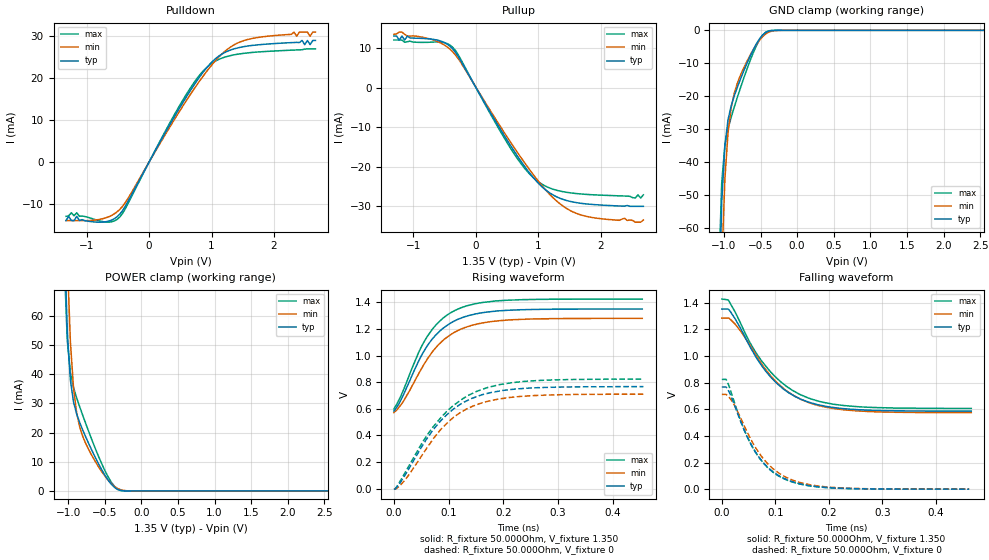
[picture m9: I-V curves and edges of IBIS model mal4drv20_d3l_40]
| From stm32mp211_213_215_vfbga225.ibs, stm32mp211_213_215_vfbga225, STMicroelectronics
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[Model] mal4drv20_d3l_40
Model_type   I/O
Polarity   Non-Inverting
Enable   Active-High
C_comp   1.902pF   1.872pF   1.915pF
C_comp_pullup   928.637fF   913.380fF   944.342fF
C_comp_pulldown   824.069fF   818.585fF   846.427fF
Vinh = 805.000mV
Vinl = 545.000mV
Vmeas = 675.000mV
Vref = 675.000mV
Rref = 50Ohms
Cref = 0pF
[Model Spec]
Vinh   805.000mV   772.000mV   855.000mV
Vinl   545.000mV   512.000mV   595.000mV
Vmeas   675.000mV   642.000mV   725.000mV
Vref   675.000mV   642.000mV   725.000mV
D_overshoot_ampl_h 0.4 NA   NA
D_overshoot_ampl_l 0.4 NA   NA
D_overshoot_area_l 110.000m NA   NA
D_overshoot_area_h 110.000m NA   NA
[Temperature Range]   25.000   125.000   -40.000
[Voltage Range]   1.350V   1.283V   1.425V
[GND Clamp Reference]   0.00V   0.00V   0.00V
[C Comp Corner]
| variable   typ   min   max
C_comp   1.902pF   1.872pF   1.915pF
C_comp_pullup   928.637fF   913.380fF   944.342fF
C_comp_pulldown   824.069fF   818.585fF   846.427fF
[Pulldown Reference]   0.00V   0.00V   0.00V
[POWER Clamp Reference]   1.350V   1.283V   1.425V
[Pullup Reference]   1.350V   1.283V   1.425V
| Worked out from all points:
|   slope of the pulldown table from 0 to 0.203 V, typ, clamps not added: 36.8 ohm
|   slope of the pullup table from 0 to 0.203 V, typ, clamps not added: 36.7 ohm
|   GND clamp passes 1 mA (typ) near -0.45 V on its own axis
|   POWER clamp passes 1 mA (typ) near -0.35 V on its own axis
|   rising waveform, R_fixture 50.000Ohm, V_fixture 1.350: 20-80 % time 66.2ps typ, 71.6ps min, 64ps max; typ from 0.584 V to 1.35 V
|   rising waveform, R_fixture 50.000Ohm, V_fixture 0: 20-80 % time 86.1ps typ, 86.2ps min, 93.2ps max; typ from -0.004 V to 0.767 V
|   falling waveform, R_fixture 50.000Ohm, V_fixture 1.350: 20-80 % time 83.5ps typ, 86.2ps min, 88.4ps max; typ from 1.35 V to 0.586 V
|   falling waveform, R_fixture 50.000Ohm, V_fixture 0: 20-80 % time 63.3ps typ, 68.1ps min, 62ps max; typ from 0.767 V to 0 V
[GND Clamp]
-1.332V   -728mA     -688mA     -718.9mA
-1.074V   -89.22mA   -115mA     -76.03mA
-1.031V   -52.27mA   -71.45mA   -46.39mA
-988mV    -34.98mA   -45.32mA   -35.1mA
-945mV    -27.21mA   -31.15mA   -29.98mA
-902mV    -22.97mA   -23.56mA   -26.45mA
-859.1mV  -19.9mA    -19.1mA    -23.3mA
-773.2mV  -14.75mA   -13.57mA   -17.39mA
-601.4mV  -5.967mA   -5.934mA   -6.902mA
-429.5mV  -634uA     -1.09mA    -554.5uA
-214.8mV  -1.1uA     -11.75uA   -194.3nA
2.663V    35.59nA    706.2nA    31.73nA
[Power Clamp]
-1.313V   833mA      802.3mA    823.6mA
-1.055V   90.5mA     128mA      79.41mA
-1.012V   54.31mA    79.78mA    51.52mA
-969.5mV  37.92mA    51.03mA    40.54mA
-926.6mV  30.49mA    35.21mA    35.43mA
-883.6mV  26.34mA    26.67mA    31.87mA
-840.7mV  23.31mA    21.76mA    28.71mA
-754.8mV  18.2mA     15.96mA    22.74mA
-583mV    9.188mA    8.193mA    11.73mA
-454.1mV  3.709mA    3.692mA    4.83mA
-325.2mV  504.5uA    850uA      638.6uA
2.682V    -27.23nA   -687.9nA   -20.2nA
[Pulldown]
-1.332V   -14mA      -14mA      -13mA
-1.16V    -13mA      -14mA      -12.14mA
-730.2mV  -14.35mA   -13.5mA    -14.29mA
-472.5mV  -12.5mA    -11.37mA   -13.18mA
515.5mV   13.58mA    12.77mA    14.16mA
988mV     23.6mA     22.88mA    23.38mA
1.246V    26.38mA    26.82mA    25.17mA
1.503V    27.49mA    28.9mA     25.9mA
2.32V     28.51mA    31mA       26.7mA
2.534V    29mA       31mA       27mA
2.577V    28mA       30mA       27mA
2.663V    29mA       31mA       27mA
[Pullup]
-1.313V   13mA       13.44mA    12mA
-1.227V   12mA       14mA       12mA
-1.184V   13mA       14mA       12mA
-1.141V   12mA       13.44mA    11.43mA
-711.8mV  12.23mA    12.15mA    11.45mA
-368.2mV  9.7mA      8.964mA    10.11mA
576.8mV   -15.19mA   -14.31mA   -15.87mA
834.5mV   -21.08mA   -20.19mA   -21.39mA
1.049V    -24.92mA   -24.6mA    -24.32mA
1.35V     -27.99mA   -29.4mA    -26.16mA
1.651V    -29.16mA   -32.01mA   -26.83mA
2.682V    -30mA      -33.44mA   -27.1mA
[Ramp]
R_load=50.000Ohm
dV/dt_r   459.300mV/77.000ps  424.798mV/80.500ps  492.900mV/79.500ps
dV/dt_f   459.300mV/74.000ps  424.799mV/78.000ps  492.900mV/76.000ps
[Rising waveform]
R_fixture=50.000Ohm
V_fixture=1.350
V_fixture_min=1.283
V_fixture_max=1.425
0s        584mV      572mV      600mV
7ps       623mV      599mV      648mV
18ps      710mV      661mV      747mV
43ps      941mV      847mV      1.004V
60ps      1.067V     968mV      1.138V
85ps      1.189V     1.096V     1.265V
118ps     1.275V     1.191V     1.352V
157ps     1.319V     1.242V     1.396V
209ps     1.341V     1.268V     1.417V
454ps     1.35V      1.28V      1.425V
[Rising waveform]
R_fixture=50.000Ohm
V_fixture=0
0s        -3.75mV    -1.041mV   -2.686mV
8ps       24.81mV    11.82mV    33.05mV
21ps      106mV      69.71mV    126mV
55ps      342mV      274mV      367mV
81ps      489mV      422mV      512mV
119ps     628mV      566mV      657mV
151ps     691mV      631mV      731mV
194ps     735mV      675mV      783mV
243ps     755mV      696mV      808mV
456ps     767mV      710mV      823mV
[Falling waveform]
R_fixture=50.000Ohm
V_fixture=1.350
V_fixture_min=1.283
V_fixture_max=1.425
0s        1.352V     1.284V     1.427V
12ps      1.352V     1.284V     1.421V
27ps      1.265V     1.229V     1.312V
53ps      1.066V     1.078V     1.097V
84ps      876mV      887mV      913mV
117ps     746mV      750mV      784mV
148ps     674mV      673mV      707mV
190ps     625mV      619mV      651mV
253ps     597mV      588mV      619mV
466ps     586mV      574mV      606mV
[Falling waveform]
R_fixture=50.000Ohm
V_fixture=0
0s        767mV      711mV      824mV
10ps      756mV      705mV      808mV
24ps      627mV      627mV      645mV
39ps      469mV      500mV      475mV
62ps      283mV      319mV      282mV
88ps      155mV      182mV      152mV
115ps     82.81mV    100mV      79.52mV
149ps     37.23mV    46.31mV    35.36mV
212ps     8.345mV    11.46mV    7.822mV
462ps     18.42uV    61.37uV    15.94uV
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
